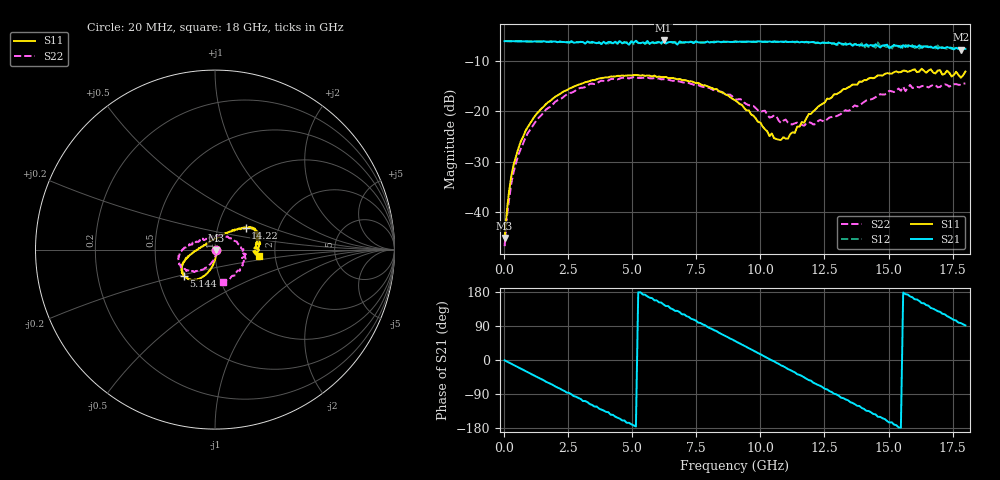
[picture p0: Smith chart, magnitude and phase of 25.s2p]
!Agilent Technologies,N5230A,US43500223,A.07.50.48
!Agilent N5230A: A.07.50.48
!Date: Monday, January 11, 2016 16:38:39
!Correction: S11(Full 2 Port(1,2))
!S21(Full 2 Port(1,2))
!S12(Full 2 Port(1,2))
!S22(Full 2 Port(1,2))
!S2P File: Measurements: S11, S21, S12, S22:
# Hz S  dB  R 50
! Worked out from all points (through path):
!   201 points, 20 MHz to 18 GHz, reference 50 ohm
!   highest |S21| = -6.03 dB at 6.223 GHz (marker M1); lowest = -7.8 dB at 17.82 GHz (marker M2)
!   group delay of S21, straight-line fit = 97.1 ps
!   lowest |S11| = -45.1 dB at 20 MHz (marker M3), VSWR 1.01, Z = 50.5 - j0.144 ohm
!   |S11| at or under -10 dB: start of sweep to end of sweep
!   |S22| runs from -46.7 to -13.3 dB; largest |S21 - S12| = 0.047
!   S11 on the Smith chart (normalised r, x): 20 MHz: 1.01, -0.00; 5.144 GHz: 0.68, -0.21; 14.22 GHz: 1.36, +0.35; 18 GHz: 1.64, -0.13
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2e7  -45.08 -14.9  -6.16 -0.9  -6.15 -0.8  -46.72 -26.5
1.099e8  -39.77 -52.1  -6.16 -4.0  -6.17 -4.0  -40.89 -50.3
2.897e8  -32.59 -72.1  -6.18 -10.2  -6.18 -10.3  -34.04 -74.4
8.291e8  -23.98 -91.5  -6.20 -29.0  -6.21 -29.1  -25.28 -96.5
1.9978e9  -17.14 -108.2  -6.23 -69.8  -6.24 -69.5  -18.14 -119.7
3.0766e9  -14.48 -119.9  -6.34 -108.4  -6.31 -107.4  -15.38 -134.0
4.0655e9  -13.33 -129.5  -6.32 -137.7  -6.61 -139.5  -13.98 -147.6
5.1443e9  -12.86 -140.1  -6.10 -175.5  -6.08 -174.4  -13.25 -158.0
6.0433e9  -13.15 -148.0  -6.34 152.2  -6.28 150.7  -13.58 -167.2
6.2231e9  -13.27 -149.5  -6.03 146.5  -6.24 147.0  -13.68 -169.6
7.5716e9  -14.42 -158.2  -6.40 98.9  -6.36 99.2  -14.84 179.7
9.01e9  -17.84 -170.6  -6.28 50.2  -6.23 49.3  -17.71 167.4
9.909e9  -22.15 169.3  -6.19 18.4  -6.26 17.5  -19.85 154.1
1.07181e10  -25.67 126.8  -6.31 -10.2  -6.28 -11.5  -21.92 139.0
1.20666e10  -20.03 59.5  -6.33 -59.8  -6.37 -60.4  -22.66 90.3
1.33252e10  -15.61 41.8  -6.85 -104.0  -6.57 -104.5  -19.83 44.7
1.42242e10  -13.55 35.8  -7.11 -134.6  -7.34 -139.9  -17.78 20.0
1.50333e10  -12.55 29.7  -7.55 -165.2  -7.21 -166.7  -15.98 0.7
1.58424e10  -12.08 25.7  -7.11 167.6  -6.64 168.5  -14.83 -18.4
1.6202e10  -12.19 21.4  -6.96 155.6  -7.63 152.6  -15.32 -26.6
1.78202e10  -13.40 -2.6  -7.82 97.6  -7.63 93.9  -14.80 -70.4
1.8e10  -12.18 -8.8  -7.67 91.4  -7.64 87.8  -14.51 -75.8
